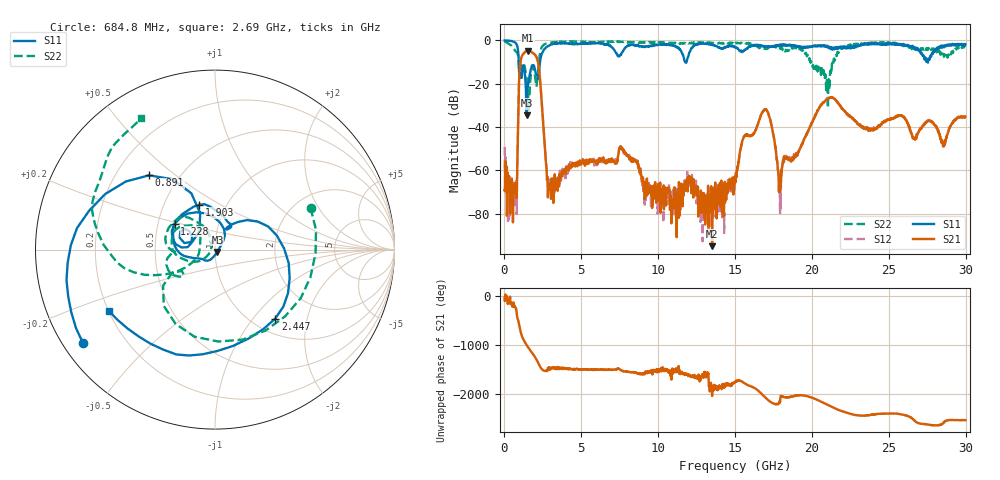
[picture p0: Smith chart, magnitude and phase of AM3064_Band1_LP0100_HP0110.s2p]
# Hz S DB R 50.0
!freq dBS11 angS11 dBS21 angS21 dBS12 angS12 dBS22 angS22
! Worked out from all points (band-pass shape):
!   1600 points, 10 MHz to 29.98 GHz, reference 50 ohm
!   highest |S21| = -4.73 dB at 1.528 GHz (marker M1); lowest = -95.0 dB at 13.51 GHz (marker M2)
!   |S21| within 3 dB of the highest: 1.109 GHz to 2.086 GHz (977 MHz wide, 61.2 % of centre)
!   lowest |S11| = -34.7 dB at 1.435 GHz (marker M3), VSWR 1.04, Z = 51.4 - j1.29 ohm
!   |S11| at or under -10 dB: 931.5 MHz to 2.312 GHz (1.381 GHz wide, 85.1 % of centre); 11.75 GHz to 11.84 GHz (89.84 MHz wide, 0.762 % of centre); 27.52319 GHz to 27.55115 GHz (27.96 MHz wide, 0.102 % of centre)
!   |S22| runs from -32.5 to -0.4 dB; largest |S21 - S12| = 0.0087
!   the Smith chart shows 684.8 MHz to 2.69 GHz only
!   S11 on the Smith chart (normalised r, x): 684.8 MHz: 0.06, -0.32; 891 MHz: 0.34, +0.41; 1.228 GHz: 0.61, +0.19; 1.903 GHz: 0.75, +0.40; 2.447 GHz: 1.26, -1.30; 2.69 GHz: 0.20, -0.26
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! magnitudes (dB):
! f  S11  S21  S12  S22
! 10 MHz  0.0  -69.2  -49.2  -0.4
! 291.2 MHz  -0.1  -62.9  -82.1  -1.6
! 684.8 MHz  -0.9  -65.9  -66.5  -4.7
! 891 MHz  -5.1  -35.2  -35.3  -7.5
! 1.228 GHz  -11.5  -6.2  -6.2  -10.9
! 1.435 GHz  -34.7  -4.9  -4.8  -17.4
! 1.528 GHz  -21.2  -4.7  -4.7  -22.6
! 1.903 GHz  -11.5  -6.1  -6.1  -12.6
! 2.447 GHz  -5.8  -30.8  -30.7  -2.9
! 2.69 GHz  -3.3  -55.6  -55.7  -1.5
! 2.972 GHz  -2.1  -67.8  -66.0  -1.1
! 5.015 GHz  -1.5  -56.4  -55.7  -0.8
! 7.62 GHz  -6.0  -49.8  -49.2  -0.7
! 10 GHz  -2.0  -74.1  -73.8  -1.0
! 13.51 GHz  -2.0  -95.0  -70.3  -1.2
! 15 GHz  -3.2  -63.1  -64.6  -1.5
! 16.88 GHz  -3.0  -32.3  -32.0  -3.7
! 17.91 GHz  -1.9  -69.3  -75.5  -3.4
! 19.99 GHz  -3.1  -38.1  -38.1  -11.2
! 25 GHz  -1.4  -36.6  -36.4  -1.2
! 28.56 GHz  -2.6  -48.3  -48.6  -6.6
! 29.98 GHz  -1.8  -35.1  -35.4  -2.8
